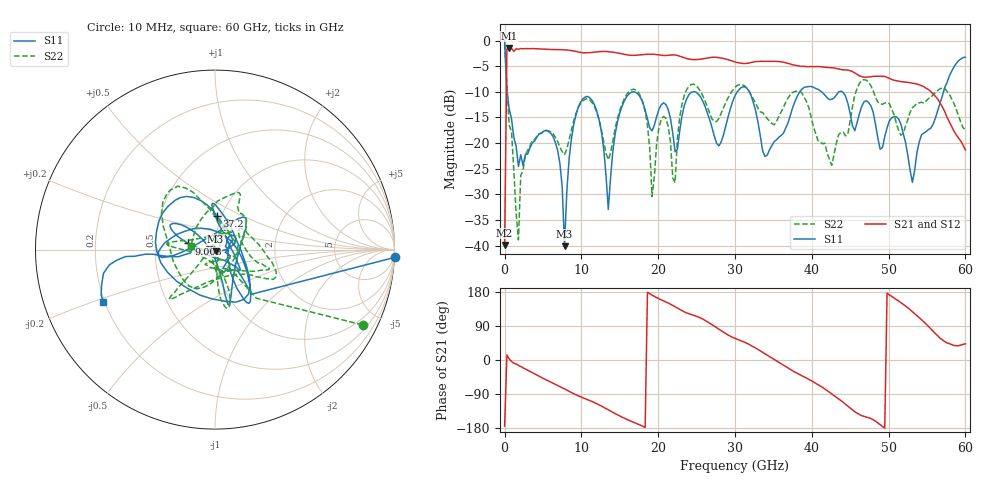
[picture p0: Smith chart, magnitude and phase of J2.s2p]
!Keysight Technologies,N5227A,US51270214,A.10.65.11
!Date: Thursday, October 15, 2020 08:05:17
!Correction: S11(Full 2 Port(1,2))
!S21(Full 2 Port(1,2))
!S12(Full 2 Port(1,2))
!S22(Full 2 Port(1,2))
!S2P File: Measurements: S11, S21, S12, S22:
# Hz S  dB  R 50
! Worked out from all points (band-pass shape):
!   201 points, 10 MHz to 60 GHz, reference 50 ohm
!   highest |S21| = -1.45 dB at 609.9 MHz (marker M1); lowest = -39.9 dB at 10 MHz (marker M2)
!   |S21| within 3 dB of the highest: 288.2 MHz to 30.88 GHz (30.59 GHz wide, 196 % of centre); 31.59 GHz to 36.88 GHz (5.293 GHz wide, 15.5 % of centre)
!   lowest |S11| = -40.1 dB at 7.809 GHz (marker M3), VSWR 1.02, Z = 50.3 - j0.925 ohm
!   |S11| at or under -10 dB: 322.7 MHz to 16.76 GHz (16.44 GHz wide, 192 % of centre); 16.84 GHz to 24.54 GHz (7.703 GHz wide, 37.2 % of centre); 43.93 GHz to 57.15 GHz (13.22 GHz wide, 26.2 % of centre)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
!   |S22| runs from -38.9 to -0.7 dB; largest |S21 - S12| = 0.1
!   S11 on the Smith chart (normalised r, x): 10 MHz: -1, -46; 9.008 GHz: 0.74, +0.05; 37.2 GHz: 0.96, +0.37; 60 GHz: 0.19, -0.22
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1e7  0.01 -2.5  -39.89 -174.6  -41.15 -176.1  -0.70 -27.0
3.0995e8  -9.85 -50.5  -1.68 13.4  -2.16 19.8  -8.98 -49.6
6.099e8  -13.37 -45.6  -1.45 2.8  -1.37 6.8  -16.54 -51.4
1.8097e9  -24.58 -15.1  -1.71 -14.1  -1.61 -13.6  -38.90 106.7
2.70955e9  -22.22 30.4  -1.57 -23.9  -1.54 -23.7  -22.37 80.6
6.30895e9  -18.71 18.9  -1.76 -61.2  -1.75 -61.2  -18.21 52.6
7.8087e9  -40.13 -68.9  -1.82 -76.4  -1.81 -76.4  -22.27 106.8
9.0085e9  -16.37 167.0  -2.04 -89.0  -2.05 -89.0  -15.66 161.7
1.02083e10  -11.37 154.9  -2.39 -99.6  -2.38 -99.7  -11.72 171.7
1.350775e10  -32.95 -154.7  -2.18 -131.5  -2.19 -131.5  -23.26 -122.8
1.56074e10  -11.74 -77.4  -2.70 -153.7  -2.71 -153.7  -11.31 -72.2
1.8007e10  -12.12 -68.2  -2.76 -174.9  -2.77 -174.9  -12.04 -84.4
1.92068e10  -17.62 -9.8  -2.67 171.3  -2.69 171.2  -30.45 -52.3
2.010665e10  -13.42 36.8  -2.81 161.6  -2.83 161.6  -16.99 65.6
2.22063e10  -21.68 98.3  -2.83 140.5  -2.84 140.5  -27.75 -162.7
2.370605e10  -11.44 -171.4  -3.51 124.2  -3.53 124.3  -9.60 -133.3
3.0005e10  -10.75 -47.3  -4.18 57.0  -4.21 57.0  -9.15 -28.2
3.72038e10  -14.63 86.3  -4.59 -25.1  -4.60 -25.1  -10.59 -18.3
4.02033e10  -9.12 153.3  -5.09 -57.7  -5.10 -58.0  -16.73 -52.9
5.010165e10  -15.69 -34.7  -7.39 171.8  -7.41 172.3  -12.32 -115.1
5.310115e10  -27.67 -114.3  -8.34 127.3  -8.35 127.4  -13.10 37.3
6e10  -3.27 -154.8  -21.37 42.9  -21.23 43.0  -17.39 170.3
